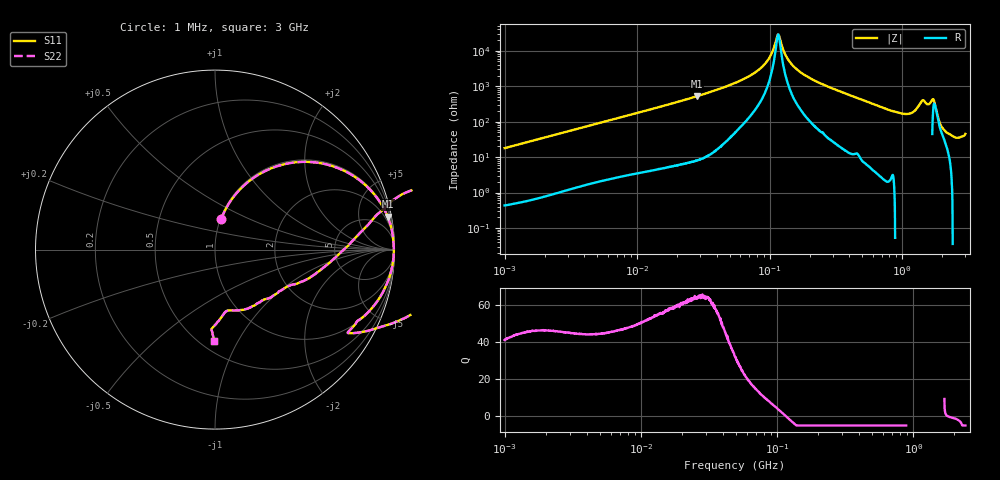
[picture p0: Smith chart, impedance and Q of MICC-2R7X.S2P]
!s-Parameter Generated by FASTRON Sdn. Bhd.
!FASTRON P/N : MICC-2R7X
!Keysight Technologies,E4991B,MY54100416,A.01.15
!Date: Fri Aug 28 09:42:10 2026
!Version  : Rev00 Fri Aug 28 09:42:10 2026
!Data & Calibration Information:
!PortZ  Port1:50+j0  Port2:50+j0
!When reading, reference impedance value at option line is always used.
!Remarks : This data is being provided solely for informational purposes.
!Freq	S11	S21	S12	S22
# Hz S dB R 50
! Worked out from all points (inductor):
!   1601 points, 1 MHz to 3 GHz, reference 50 ohm
!   read as one part in series: L = 2.84 uH near 1.041 MHz
!   highest Q = 64.6 at 28.29 MHz (marker M1), where L = 2.93 uH
!   self-resonance near 116 MHz
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1000000  -15.13 78.5  -0.17 -10.1  -0.17 -10.1  -15.13 78.5
3804036  -5.16 55.2  -1.71 -33.5  -1.71 -33.5  -5.16 55.2
6934716  -2.33 38.9  -4.04 -49.9  -4.04 -49.9  -2.33 38.9
1.447069e7  -0.67 21.3  -8.80 -67.7  -8.80 -67.7  -0.67 21.3
2.829425e7  -0.18 10.8  -14.51 -78.3  -14.51 -78.3  -0.18 10.8
5.477226e7  -0.06 4.6  -21.87 -83.1  -21.87 -83.1  -0.06 4.6
8.98892e7  -0.03 1.5  -31.76 -80.5  -31.76 -80.5  -0.03 1.5
1.013595e8  -0.03 0.8  -37.17 -74.5  -37.17 -74.5  -0.03 0.8
1.160221e8  -0.03 0.0  -49.22 -0.0  -49.22 -0.0  -0.03 0.0
1.314834e8  -0.03 -0.7  -37.73 73.7  -37.73 73.7  -0.03 -0.7
1.445978e8  -0.03 -1.3  -32.97 79.7  -32.97 79.7  -0.03 -1.3
2.083556e8  -0.05 -3.6  -23.97 83.1  -23.97 83.1  -0.05 -3.6
7.925923e8  -0.89 -24.9  -7.52 64.6  -7.52 64.6  -0.89 -24.9
1.097256e9  -1.15 -32.1  -5.49 61.0  -5.49 61.0  -1.15 -32.1
1.281378e9  0.11 -25.4  -7.08 78.9  -7.08 78.9  0.11 -25.4
1.388188e9  1.73 -13.8  -9.26 122.4  -9.26 122.4  1.73 -13.8
1.503902e9  2.78 7.7  -7.75 -153.2  -7.75 -153.2  2.78 7.7
1.596974e9  1.69 16.8  -8.24 -114.9  -8.24 -114.9  1.69 16.8
1.730092e9  -1.51 8.0  -13.77 -34.9  -13.77 -34.9  -1.51 8.0
1.990301e9  -6.95 -27.8  -3.90 19.1  -3.90 19.1  -6.95 -27.8
2.568929e9  -9.20 -77.9  -0.11 20.1  -0.11 20.1  -9.20 -77.9
3e9  -5.85 -90.6  1.04 26.9  1.04 26.9  -5.85 -90.6
